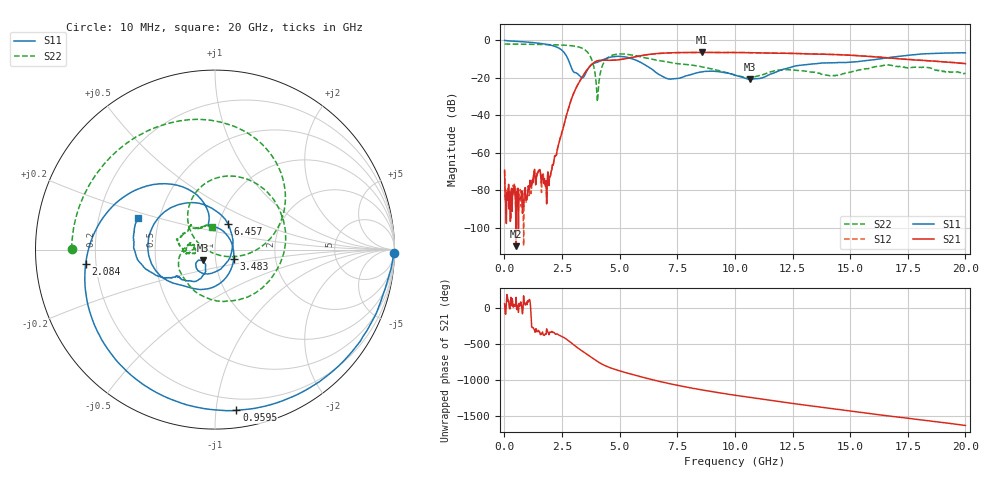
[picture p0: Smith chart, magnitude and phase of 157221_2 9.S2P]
!  2-Port S-parameters saved by WinCal
! VAR MeasName=S-Parameters (CALIBRATED_DATA) read from VNA (N5242A)
! VAR MeasDate=2015-5-26 16:47:47
! VAR NAME=157221_2 9
! VAR FILENAME=157221_2 9.S2P
! VAR DATE=2015-5-26 16:47:47
! VAR PHYS_PORTS=1,2
# Hz S DB R 50
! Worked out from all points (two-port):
!   801 points, 10 MHz to 20 GHz, reference 50 ohm
!   highest |S21| = -6.41 dB at 8.581 GHz (marker M1); lowest = -109.9 dB at 509.8 MHz (marker M2)
!   |S21| within 3 dB of the highest: 5.403 GHz to 16.69 GHz (11.28 GHz wide, 102 % of centre)
!   lowest |S11| = -20.8 dB at 10.65 GHz (marker M3), VSWR 1.20, Z = 43.3 - j5.27 ohm
!   |S11| at or under -10 dB: 2.762 GHz to 4.348 GHz (1.586 GHz wide, 44.6 % of centre); 5.588 GHz to 16.21 GHz (10.62 GHz wide, 97.5 % of centre)
!   |S22| runs from -32.7 to -2.0 dB; largest |S21 - S12| = 0.01
!   S11 on the Smith chart (normalised r, x): 10 MHz: open; 959.5 MHz: 0.12, -1.14; 2.084 GHz: 0.16, -0.05; 3.483 GHz: 1.23, -0.12; 6.457 GHz: 1.11, +0.33; 20 GHz: 0.38, +0.17
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1e7  -0.04 -1.1  -69.32 61.6  -69.39 -101.0  -1.96 179.7
5.0975e8  -0.50 -45.2  -109.90 152.3  -87.67 12.4  -1.99 167.7
9.59525e8  -0.88 -82.4  -85.49 84.4  -84.48 82.5  -2.05 156.6
1.484262e9  -1.50 -123.7  -69.39 53.8  -69.64 43.2  -2.15 143.0
1.859075e9  -2.18 -153.9  -76.01 55.6  -78.74 41.7  -2.24 132.3
2.083962e9  -2.79 -173.8  -66.64 29.3  -66.45 26.7  -2.31 125.3
2.583712e9  -6.35 130.4  -45.30 -45.5  -45.23 -45.8  -2.55 106.9
3.358325e9  -19.93 32.7  -19.95 130.8  -19.92 130.5  -4.09 61.6
3.483262e9  -18.74 -25.7  -17.54 103.3  -17.50 103.0  -4.95 49.7
3.783112e9  -13.00 -101.8  -12.90 37.0  -12.88 36.6  -10.08 11.2
4.032988e9  -11.64 -128.4  -10.95 -17.2  -10.95 -17.4  -32.74 -96.2
4.632688e9  -8.86 -166.4  -10.63 -110.0  -10.61 -110.4  -8.16 92.2
5.532238e9  -9.75 130.3  -9.08 163.3  -9.08 162.8  -7.80 16.4
6.456775e9  -15.86 63.0  -7.22 86.1  -7.26 85.8  -10.18 -64.1
6.681662e9  -17.99 42.3  -6.99 68.5  -7.00 68.4  -10.70 -81.8
8.580712e9  -16.75 -111.0  -6.41 -53.3  -6.41 -53.5  -14.15 -171.6
1.0005e10  -18.55 -146.5  -6.50 -126.9  -6.50 -127.3  -18.54 173.5
1.065468e10  -20.80 -138.6  -6.59 -158.3  -6.57 -158.5  -19.54 -172.6
1.335332e10  -12.58 -132.1  -7.29 83.2  -7.21 82.9  -16.93 164.5
1.497751e10  -11.62 -145.9  -7.93 14.7  -7.90 14.1  -16.94 -173.7
1.667666e10  -9.19 -154.8  -9.38 -55.0  -9.39 -55.4  -13.16 164.9
2e10  -6.62 157.7  -12.42 173.7  -12.47 172.2  -17.79 96.5
